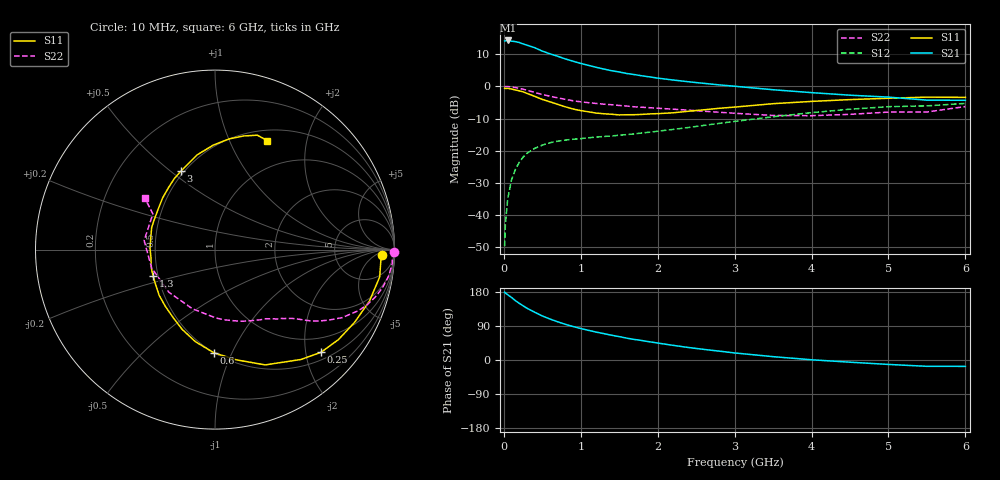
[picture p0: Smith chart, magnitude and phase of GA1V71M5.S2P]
! Infineon Technologies  Discrete & RF Semiconductors
! BF775
! Si NPN RF Bipolar Junction Transistor in SOT23
! VCE = 1.75 V  IC = 1.5 mA
! Common Emitter S-Parameters:  May  1996
# GHz  S  MA  R  50
!  f  S11  S21  S12  S22
! GHz  MAG  ANG  MAG  ANG  MAG  ANG  MAG  ANG
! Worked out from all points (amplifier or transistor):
!   36 points, 10 MHz to 6 GHz, reference 50 ohm
!   highest |S21| = 14.2 dB at 50 MHz (marker M1)
!   |S21| within 3 dB of that: start of sweep to 471.6 MHz
!   unconditionally stable (mu >= 1): 1.238 GHz to end of sweep
!   at 250 MHz: K = 0.25, MSG = 17.6 dB, |S12| = -22.0 dB
!   at 1.4 GHz: K = 1.08, MAG = 8.4 dB, |S12| = -15.4 dB
!   at 6 GHz: K = 1.04, MAG = -0.8 dB, |S12| = -5.3 dB
!   S11 on the Smith chart (normalised r, x): 10 MHz: 23, -11; 250 MHz: 0.65, -2.31; 600 MHz: 0.50, -0.85; 1.3 GHz: 0.47, -0.16; 3 GHz: 0.48, +0.54; 6 GHz: 0.63, +1.39
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0.01  0.9327 -2.0  5.051 178.8  0.0033 93.0  0.9987 -0.8
0.02  0.926 -3.8  5.069 176.8  0.0072 88.7  0.9883 -1.7
0.05  0.9302 -9.4  5.152 172.3  0.0178 85.6  0.991 -4.5
0.1  0.9072 -18.4  5.028 165.0  0.0354 79.2  0.9784 -8.8
0.15  0.8771 -27.5  4.938 156.6  0.0513 73.4  0.9559 -13.0
0.2  0.8512 -36.1  4.794 149.7  0.0659 68.6  0.9298 -16.7
0.25  0.8223 -44.1  4.552 143.1  0.0795 64.1  0.9008 -20.0
0.3  0.7771 -52.0  4.356 136.7  0.0911 60.6  0.8704 -22.9
0.4  0.7005 -66.5  3.981 126.1  0.1089 53.4  0.8042 -28.1
0.5  0.6257 -79.0  3.523 116.2  0.122 48.2  0.7458 -31.8
0.6  0.5745 -90.7  3.193 108.1  0.1331 44.3  0.7023 -34.5
0.8  0.4805 -112.4  2.662 94.1  0.1464 39.2  0.6278 -38.6
0.9  0.4444 -121.8  2.451 88.3  0.1508 38.1  0.5967 -40.3
1.1  0.402 -140.8  2.113 78.3  0.1589 36.5  0.5569 -43.5
1.3  0.3753 -156.9  1.853 69.6  0.1666 35.9  0.5284 -46.5
1.7  0.3625 172.0  1.52 54.2  0.1826 37.9  0.4803 -53.3
2.2  0.3882 144.8  1.253 38.7  0.2143 39.8  0.4419 -63.9
3  0.4761 113.6  1.003 18.6  0.2852 38.9  0.3816 -89.0
3.5  0.5375 100.6  0.885 8.8  0.3368 35.1  0.3529 -110.9
4.5  0.6222 82.6  0.728 -5.8  0.4414 23.2  0.3672 -163.7
5.5  0.6796 69.7  0.61 -16.7  0.4973 7.7  0.3992 150.1
6  0.6738 64.4  0.607 -16.8  0.5428 3.4  0.4856 143.7
